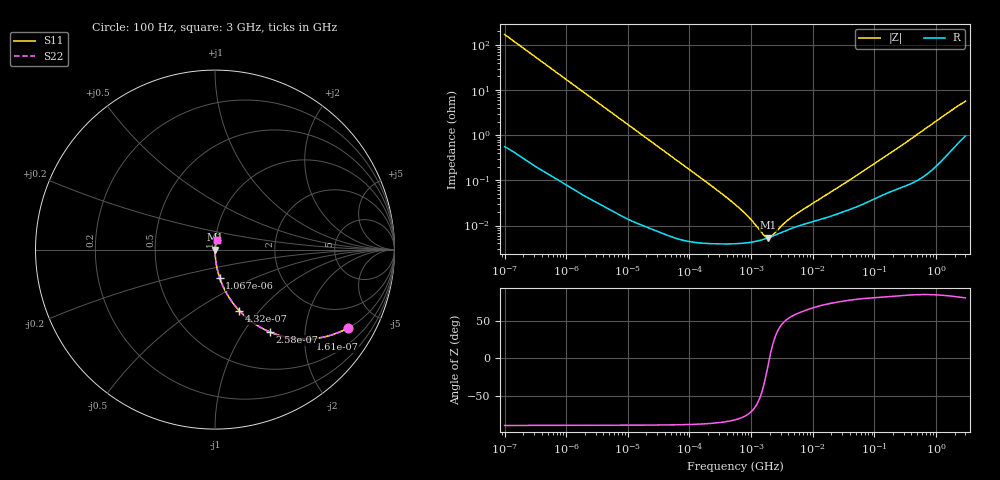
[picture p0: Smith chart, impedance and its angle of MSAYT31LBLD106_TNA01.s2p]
! MSAYT31LBLD106_TNA01  S-PARAMETER MODEL  ( Standard Model )
! Model Generated by TAIYO YUDEN Corporation (http://www.ty-top.com)
! Version 1.0
! TAIYO YUDEN Control No. 220601
! Copyright(c) 2012 TAIYO YUDEN CO.,LTD. All Rights Reserved.
! Product Description (link to TY-COMPAS)
! https://ds.yuden.co.jp/TYCOMPAS/or/detail?pn=MSAYT31LBLD106KTNA01&u=M
! Products Name : Multilayer Ceramic Capacitors
! Characteristics :
!  Capacitance : 10 [uF] , Rated Voltage : 25 [V] , TCC : X5R
!  Case Size : 3.2 x 1.6 / 0.126 x 0.063 [mm/inch] , Thickness : 1.6 / 0.063 [mm/inch]
!  (Conditions: Temperature = 25 [degC] , DC Bias Voltage = 0 [V])
! External Node Assignments :
!  1  o---| |---o  2
! GND o---------o GND
! Frequency Range : 100Hz  -  3GHz  [ 401 STEP ]
# MHZ S RI R 50
! Freq[MHz].  S11 Real  S11 Imag  S21 Real  S21 Imag  S12 Real  S12 Imag  S22 Real  S22 Imag
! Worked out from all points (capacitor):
!   401 points, 100 Hz to 3 GHz, reference 50 ohm
!   read as one part in series: C = 9.34 uF near 109 Hz
!   lowest |Z| = 5.41 mohm at 1.908 MHz (marker M1)
!   series resonance near 1.992 MHz, so ESL is about 680 pH
!   S11 on the Smith chart (normalised r, x): 100 Hz: 1.01, -3.41; 161 Hz: 1.01, -2.12; 258 Hz: 1.00, -1.32; 432 Hz: 1.00, -0.79; 1.067 kHz: 1.00, -0.32; 3 GHz: 1.02, +0.11
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0.0001  0.7428 -0.4354  0.2572 0.4354  0.2572 0.4354  0.7428 -0.4354
0.000161  0.5299 -0.4973  0.4701 0.4973  0.4701 0.4973  0.5299 -0.4973
0.000258  0.3054 -0.4587  0.6946 0.4587  0.6946 0.4587  0.3054 -0.4587
0.000432  0.1362 -0.341  0.8638 0.341  0.8638 0.341  0.1362 -0.341
0.000636  0.0683 -0.2501  0.9317 0.2501  0.9317 0.2501  0.0683 -0.2501
0.001067  0.0258 -0.1563  0.9742 0.1563  0.9742 0.1563  0.0258 -0.1563
0.001788  0.00959 -0.095  0.9904 0.095  0.9904 0.095  0.00959 -0.095
0.005476  0.0012 -0.0314  0.9988 0.0314  0.9988 0.0314  0.0012 -0.0314
0.031977  0.000101 -0.00542  0.9999 0.00542  0.9999 0.00542  0.000101 -0.00542
0.221826  4.02e-05 -0.000776  1 0.000776  1 0.000776  4.02e-05 -0.000776
0.547723  3.96e-05 -0.000293  1 0.000293  1 0.000293  3.96e-05 -0.000293
0.772864  4.08e-05 -0.000189  1 0.000189  1 0.000189  4.08e-05 -0.000189
1.188587  4.46e-05 -9.16e-05  1 9.16e-05  1 9.16e-05  4.46e-05 -9.16e-05
1.295438  4.58e-05 -7.49e-05  1 7.49e-05  1 7.49e-05  4.58e-05 -7.49e-05
1.908323  5.37e-05 -6.97e-06  0.9999 6.97e-06  0.9999 6.97e-06  5.37e-05 -6.97e-06
2.81117  6.63e-05 5.35e-05  0.9999 -5.35e-05  0.9999 -5.35e-05  6.63e-05 5.35e-05
3.198641  7.14e-05 7.29e-05  0.9999 -7.29e-05  0.9999 -7.29e-05  7.14e-05 7.29e-05
5.135543  9.19e-05 0.000146  0.9999 -0.000146  0.9999 -0.000146  9.19e-05 0.000146
9.794414  0.00012 0.000278  0.9999 -0.000278  0.9999 -0.000278  0.00012 0.000278
175.1444  0.000561 0.00384  0.9994 -0.00384  0.9994 -0.00384  0.000561 0.00384
1642.185  0.00513 0.0324  0.9949 -0.0324  0.9949 -0.0324  0.00513 0.0324
3000  0.0125 0.0547  0.9875 -0.0547  0.9875 -0.0547  0.0125 0.0547
